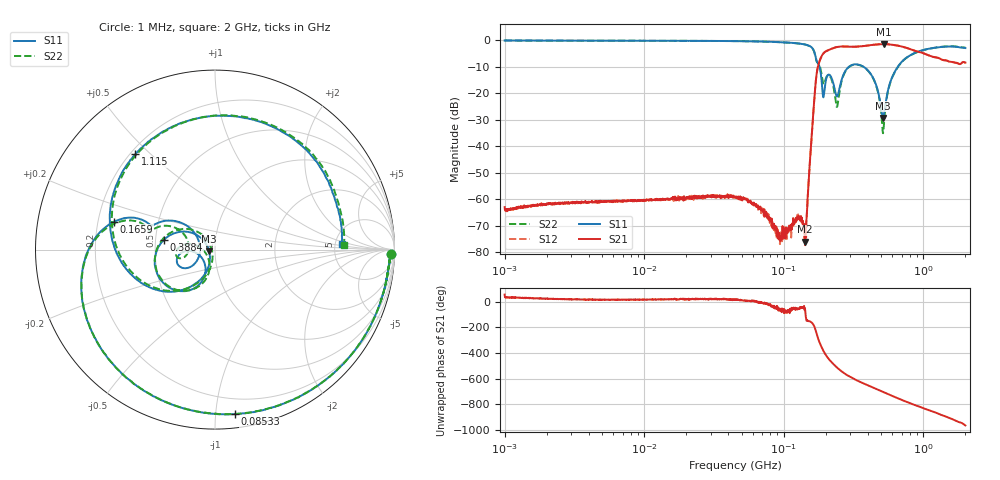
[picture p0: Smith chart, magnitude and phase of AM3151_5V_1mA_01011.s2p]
! Date/Time: Fri Jun 26 10:44:55 2020
! Network Analyzer:  Rev:
! Sweep from 1000000.0 to 2000000000.0, 1601 Points ! Power Supply: 0 V, 0 A
# HZ S DB R 50
!freq MagS11 AngS11 MagS21 AngS21 MagS12 AngS12 MagS22 AngS22
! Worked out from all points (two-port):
!   1601 points, 1 MHz to 2 GHz, reference 50 ohm
!   highest |S21| = -1.53 dB at 521.4 MHz (marker M1); lowest = -76.0 dB at 142.5 MHz (marker M2)
!   |S21| within 3 dB of the highest: 196.3 MHz to 938.2 MHz (741.9 MHz wide, 131 % of centre)
!   lowest |S11| = -29.4 dB at 514 MHz (marker M3), VSWR 1.07, Z = 46.8 - j0.826 ohm
!   |S11| at or under -10 dB: 180.2 MHz to 293.8 MHz (113.6 MHz wide, 47.9 % of centre); 371.4 MHz to 657.1 MHz (285.7 MHz wide, 55.6 % of centre)
!   |S22| runs from -35.1 to -0.1 dB; largest |S21 - S12| = 0.0088
!   S11 on the Smith chart (normalised r, x): 1 MHz: 37, -53; 85.33 MHz: 0.09, -1.12; 165.9 MHz: 0.27, +0.13; 388.4 MHz: 0.55, +0.07; 1.115 GHz: 0.22, +0.45; 2 GHz: 5.76, +0.71
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1000000  -0.16 -1.4  -62.97 55.2  -63.92 36.7  -0.15 -1.5
3555161  -0.22 -3.9  -60.99 18.0  -60.83 16.1  -0.22 -3.9
1.263916e7  -0.27 -12.6  -60.16 16.2  -60.23 17.4  -0.27 -12.6
4.493426e7  -0.40 -44.0  -59.16 13.7  -59.25 16.7  -0.41 -43.9
8.533003e7  -0.70 -83.2  -69.49 -44.6  -71.13 -38.8  -0.70 -83.1
1.425349e8  -1.69 -147.1  -76.04 -72.5  -75.07 -64.9  -1.70 -146.9
1.589914e8  -2.84 -177.2  -34.91 -163.9  -34.88 -164.0  -2.86 -176.8
1.659366e8  -4.67 164.6  -21.36 163.4  -21.35 163.3  -4.77 165.4
1.790408e8  -9.49 152.2  -8.45 51.5  -8.45 51.4  -9.05 160.2
1.913533e8  -21.40 170.2  -5.14 -18.6  -5.14 -18.6  -16.34 166.7
2.175411e8  -13.76 -171.0  -3.39 -105.8  -3.37 -105.7  -14.22 174.8
2.403627e8  -21.25 -146.0  -2.61 -152.6  -2.60 -152.6  -25.22 -147.9
2.643201e8  -13.78 -113.4  -2.43 171.0  -2.43 171.0  -14.13 -109.9
3.883688e8  -10.76 169.1  -2.15 75.0  -2.15 75.1  -10.84 165.6
4.564482e8  -16.63 142.7  -1.67 42.1  -1.69 42.0  -16.81 135.3
5.140083e8  -29.40 -164.9  -1.53 17.5  -1.53 17.5  -35.12 -168.5
5.213857e8  -28.21 -139.8  -1.53 14.4  -1.52 14.5  -31.93 -125.1
5.652395e8  -17.74 -111.2  -1.62 -2.3  -1.61 -2.3  -18.06 -106.4
7.69728e8  -6.35 -162.1  -3.05 -62.7  -3.06 -62.7  -6.43 -164.0
1.114967e9  -3.20 129.9  -5.95 -127.6  -5.93 -127.6  -3.19 126.7
1.489751e9  -2.45 72.2  -7.93 -179.8  -7.80 179.8  -2.38 69.3
2e9  -3.00 2.5  -8.48 116.6  -8.62 116.0  -2.86 2.0
